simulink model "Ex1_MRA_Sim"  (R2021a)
settings: Solver=VariableStepAuto  StartTime=0.0  StopTime=10.0  RelTol=1e-3
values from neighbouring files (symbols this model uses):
  fv = 4    [Ex1_MRA.m]
  K = 50    [Ex1_MRA.m]
  M = 2    [Ex1_MRA.m]

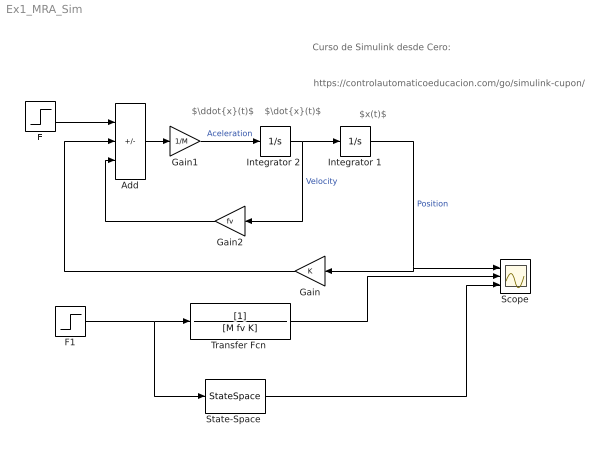
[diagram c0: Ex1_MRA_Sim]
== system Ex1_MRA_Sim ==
  note: https://controlautomaticoeducacion.com/go/simulink-cupon/
  note: Curso de Simulink desde Cero:
  note: $x(t)$
  note: $\dot{x}(t)$
  note: $\ddot{x}(t)$
  Add : Sum  Inputs=+--
  F : Step  SampleTime=0
  F1 : Step  SampleTime=0
  Gain : Gain  Gain=K
  Gain1 : Gain  Gain=1/M
  Gain2 : Gain  Gain=fv
  Integrator 1 : Integrator
  "Integrator 2 " : Integrator
  Scope : Scope  NumInputPorts=3
  "State-Space " : StateSpace  A=[0,1; -K/M, -fv/M]  B=[0;1/M]  C=[1, 0]  D=0  InitialCondition=0
  "Transfer Fcn " : TransferFcn  Denominator=[M fv K]
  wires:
  "Integrator 2 "/1 -> Gain2/1, Integrator 1/1  "Velocity"
  Integrator 1/1 -> Gain/1, Scope/1  "Position"
  Gain1/1 -> "Integrator 2 "/1  "Aceleration"
  Add/1 -> Gain1/1
  F/1 -> Add/1
  Gain/1 -> Add/2
  Gain2/1 -> Add/3
  F1/1 -> "State-Space "/1, "Transfer Fcn "/1
  "Transfer Fcn "/1 -> Scope/2
  "State-Space "/1 -> Scope/3
